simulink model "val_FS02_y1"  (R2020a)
settings: Solver=ode45  StartTime=0.0  StopTime=100  RelTol=1e-3  EnableMultiTasking=on
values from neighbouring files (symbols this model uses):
  Ts = 0.05    [init_model.m]
libraries: fuzblock x1

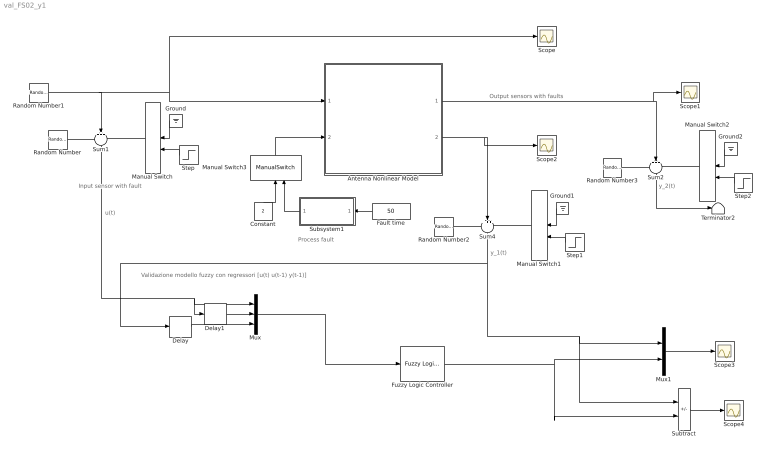
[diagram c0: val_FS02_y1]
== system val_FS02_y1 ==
  note: Validazione modello fuzzy con regressori [u(t) u(t-1) y(t-1)]
  note: u(t)
  note: Output sensors with faults
  note: Process fault
  note: Input sensor with fault
  note: y_1(t)
  note: y_2(t)
  Antenna Nonlinear Model : Subsystem
  Constant : Constant  Value=2
  Delay : Delay  DelayLength=1  SampleTime=Ts
  Delay1 : Delay  DelayLength=1  SampleTime=Ts
  Fault time : Constant  Value=50
  Fuzzy Logic Controller : fuzblock/Fuzzy Logic  Controller  FIS=FIS02  OutputSampleNumber=101  DataType=double  FuzzifiedInputs=off  RuleFiringStrengths=off  RuleOutputs=off  AggregatedOutputs=off  SimulateUsing=Interpreted execution  OutOfRangeInputValueMessage=warning  NoRuleFiredMessage=warning  EmptyOutputFuzzySetMessage=warning
  Ground : Ground
  Ground1 : Ground
  Ground2 : Ground
  Manual Switch : ManualSwitch
  Manual Switch1 : ManualSwitch  CurrentSetting=0
  Manual Switch2 : ManualSwitch
  Manual Switch3 : ManualSwitch
  Mux : Mux  Inputs=3
  Mux1 : Mux  Inputs=2
  Random Number : RandomNumber  Variance=0.0001  Seed=1  SampleTime=Ts
  Random Number1 : RandomNumber  Variance=0.1  SampleTime=10
  Random Number2 : RandomNumber  Variance=0.00001  Seed=2  SampleTime=Ts
  Random Number3 : RandomNumber  Variance=0.00001  Seed=3  SampleTime=Ts
  Scope{,1..4} (5 alike) : Scope
  Step : Step  Time=50  SampleTime=0
  Step1 : Step  Time=50  SampleTime=0
  Step2 : Step  Time=50  SampleTime=0
  Subsystem1 : Subsystem
  Subtract : Sum  Inputs=+-
  Sum1 : Sum  Inputs=+++  SaturateOnIntegerOverflow=on
  Sum2 : Sum  Inputs=+++  SaturateOnIntegerOverflow=on
  Sum4 : Sum  Inputs=+++  SaturateOnIntegerOverflow=on
  Terminator2 : Terminator
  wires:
  Random Number1/1 -> Scope/1, Antenna Nonlinear Model/1(force), Sum1/2
  Random Number/1 -> Sum1/1
  Manual Switch/1 -> Sum1/3
  Sum1/1 -> Delay1/1, Mux/1
  Ground/1 -> Manual Switch/1
  Step/1 -> Manual Switch/2
  Random Number2/1 -> Sum4/1
  Ground1/1 -> Manual Switch1/1
  Manual Switch1/1 -> Sum4/3
  Step1/1 -> Manual Switch1/2
  Antenna Nonlinear Model/2(velocity) -> Sum4/2, Scope2/1
  Random Number3/1 -> Sum2/1
  Ground2/1 -> Manual Switch2/1
  Manual Switch2/1 -> Sum2/3
  Step2/1 -> Manual Switch2/2
  Antenna Nonlinear Model/1(angle) -> Sum2/2, Scope1/1
  Sum2/1 -> Terminator2/1
  Fault time/1 -> Subsystem1/1(Fault time)
  Subsystem1/1(Fault) -> Manual Switch3/2
  Manual Switch3/1 -> Antenna Nonlinear Model/2(drag)
  Constant/1 -> Manual Switch3/1
  Delay/1 -> Mux/3
  Delay1/1 -> Mux/2
  Subtract/1 -> Scope4/1
  Mux1/1 -> Scope3/1
  Fuzzy Logic Controller/1 -> Subtract/2, Mux1/2
  Mux/1 -> Fuzzy Logic Controller/1
  Sum4/1 -> Subtract/1, Mux1/1, Delay/1

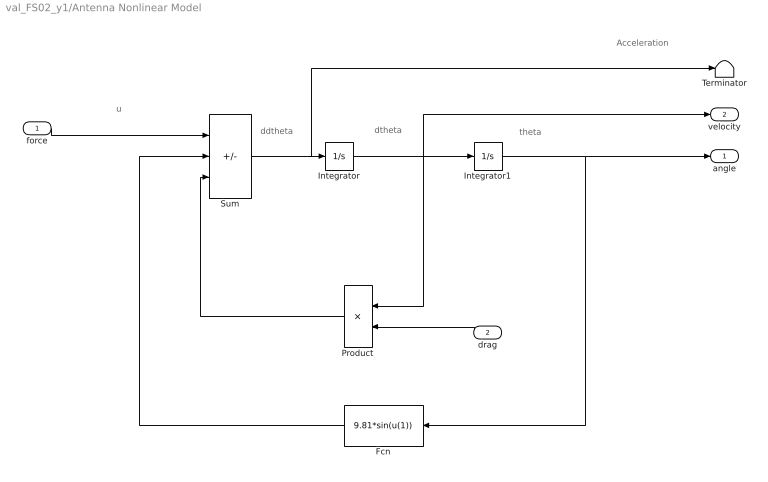
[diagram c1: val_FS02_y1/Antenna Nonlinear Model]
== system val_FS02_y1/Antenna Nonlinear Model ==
  note: Acceleration
  note: ddtheta
  note: dtheta
  note: theta
  note: u
  force : Inport
  drag : Inport  Port=2
  Fcn : Fcn  Expr=9.81*sin(u(1))
  Integrator : Integrator
  Integrator1 : Integrator  InitialCondition=(pi/180)*90
  Product : Product
  Sum : Sum  Inputs=+--  SaturateOnIntegerOverflow=on
  Terminator : Terminator
  angle : Outport
  velocity : Outport  Port=2
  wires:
  Sum/1 -> Terminator/1, Integrator/1
  Integrator/1 -> Product/1, Integrator1/1, velocity/1
  Integrator1/1 -> angle/1, Fcn/1
  Fcn/1 -> Sum/2
  Product/1 -> Sum/3
  force/1 -> Sum/1
  drag/1 -> Product/2

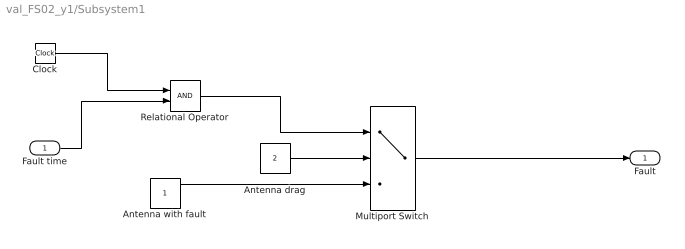
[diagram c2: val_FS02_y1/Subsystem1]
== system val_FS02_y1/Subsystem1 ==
  Fault time : Inport
  Antenna drag : Constant  Value=2
  Antenna with fault : Constant
  Clock : Clock
  Multiport Switch : MultiPortSwitch  DataPortOrder=Zero-based contiguous  Inputs=2  zeroidx=on
  Relational Operator : RelationalOperator  OutDataTypeStr=boolean  RndMeth=Simplest
  Fault : Outport
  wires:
  Clock/1 -> Relational Operator/1
  Fault time/1 -> Relational Operator/2
  Antenna drag/1 -> Multiport Switch/2
  Relational Operator/1 -> Multiport Switch/1
  Multiport Switch/1 -> Fault/1
  Antenna with fault/1 -> Multiport Switch/3
